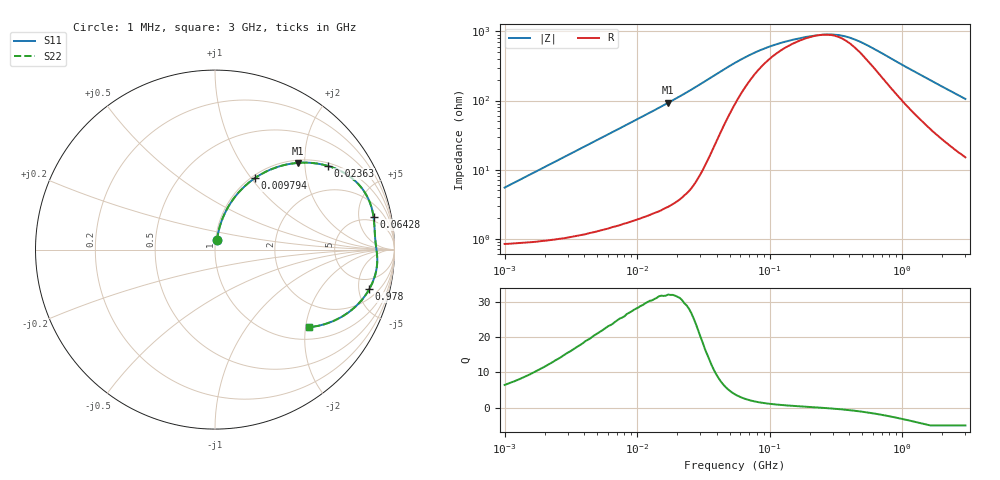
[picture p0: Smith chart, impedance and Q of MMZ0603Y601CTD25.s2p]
! S-Parameter Data Generated by TDK Corporation
! Copyright(C) 2025 TDK Corporation.
! All Rights Reserved.
! TDK P/N: MMZ0603Y601CTD25 (Chip Bead)
! Property: |Z|=600ohm at 100MHz
! Size(LxWxT): 0.6x0.3x0.3mm
! Model Type: s2p (Touchstone File Format Version 1.0)
! Frequency: DC=Yes Start=1MHz Stop=3000MHz 202points Log-sweep
! Model Generated on Feb. 6, 2025
! Terms and conditions regarding TDK Simulation Models:
! 1)This simulation model is being provided solely for informational
!  purposes. Please refer to the specifications of the products in
!  terms of detailed characteristics of such products.
! 2)In no event shall TDK Corporation of any of its subsidiaries be
!  liable for any loss or damage arising, directly or indirectly,
!  from any information contained in this simulation model, including,
!  but not limited to loss or damages arising from any inaccuracies,
!  omissions or errors in connection with such information.
! 3)Any and all copyrights on this simulation model are owned by
!  TDK Corporation.  Duplication or redistribution of this simulation
!  model without prior written permission from TDK Corporation
!  is prohibited.
! 4)This simulation model is subject to any modification or change
!  without any prior notice.
! 5)Neither TDK Corporation nor any of its subsidiaries shall make any
!  warranty, express or implied, including but not limited to the
!  correctness, implied warranties of merchantability and fitness for
!  a particular purpose with respect to this simulation models.
! 6)The use of this simulation model shall be deemed to have consented
!  to the terms and conditions hereof.
! Port Assignments:
!  1 ---@@@--- 2
! Applicable Conditions:
!  Temperature = 25 degC
!  DC Bias Current = 0 A
!  Small Signal Operation
# Hz S MA R 50
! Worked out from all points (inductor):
!   201 points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, 1 MHz to 3 GHz, reference 50 ohm
!   read as one part in series: L = 863 nH near 1.041 MHz
!   highest Q = 31.9 at 17.15 MHz (marker M1), where L = 860 nH
!   self-resonance near 248.3 MHz
!   S11 on the Smith chart (normalised r, x): 1 MHz: 1.02, +0.11; 9.794 MHz: 1.04, +1.05; 23.63 MHz: 1.09, +2.62; 64.28 MHz: 3.98, +7.77; 978 MHz: 3.09, -6.43; 3 GHz: 1.30, -2.09
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1000000  0.05434 78.1  0.9902 -3.1  0.9902 -3.1  0.05434 78.1
2055611  0.1098 78.9  0.9848 -6.3  0.9848 -6.3  0.1098 78.9
3900413  0.2035 75.2  0.968 -11.7  0.968 -11.7  0.2035 75.2
6305767  0.3161 69.1  0.9353 -18.4  0.9353 -18.4  0.3161 69.1
9794439  0.4573 60.8  0.8732 -27.2  0.8732 -27.2  0.4573 60.8
1.461624e7  0.6083 50.7  0.7747 -37.4  0.7747 -37.4  0.6083 50.7
1.71545e7  0.6697 46.2  0.7221 -42.0  0.7221 -42.0  0.6697 46.2
2.362996e7  0.7821 36.6  0.5968 -51.4  0.5968 -51.4  0.7821 36.6
3.670325e7  0.883 23.6  0.401 -61.6  0.401 -61.6  0.883 23.6
5.477226e7  0.9033 14.4  0.2569 -60.9  0.2569 -60.9  0.9033 14.4
6.428402e7  0.9018 11.7  0.2166 -57.4  0.2166 -57.4  0.9018 11.7
1.081723e8  0.895 5.7  0.1404 -38.9  0.1404 -38.9  0.895 5.7
1.49005e8  0.8948 3.3  0.1182 -25.5  0.1182 -25.5  0.8948 3.3
2.136344e8  0.8976 1.0  0.1036 -8.3  0.1036 -8.3  0.8976 1.0
2.942768e8  0.9021 -1.1  0.0997 10.4  0.0997 10.4  0.9021 -1.1
3.741707e8  0.9053 -3.0  0.1068 26.1  0.1068 26.1  0.9053 -3.0
4.951867e8  0.9069 -5.5  0.1308 41.9  0.1308 41.9  0.9069 -5.5
8.005644e8  0.8981 -11.4  0.2138 56.0  0.2138 56.0  0.8981 -11.4
9.779672e8  0.8871 -14.5  0.2626 57.5  0.2626 57.5  0.8871 -14.5
1.645649e9  0.8266 -24.6  0.4242 54.2  0.4242 54.2  0.8266 -24.6
2.266846e9  0.7591 -32.2  0.5403 48.5  0.5403 48.5  0.7591 -32.2
3e9  0.6786 -39.6  0.644 42.2  0.644 42.2  0.6786 -39.6
